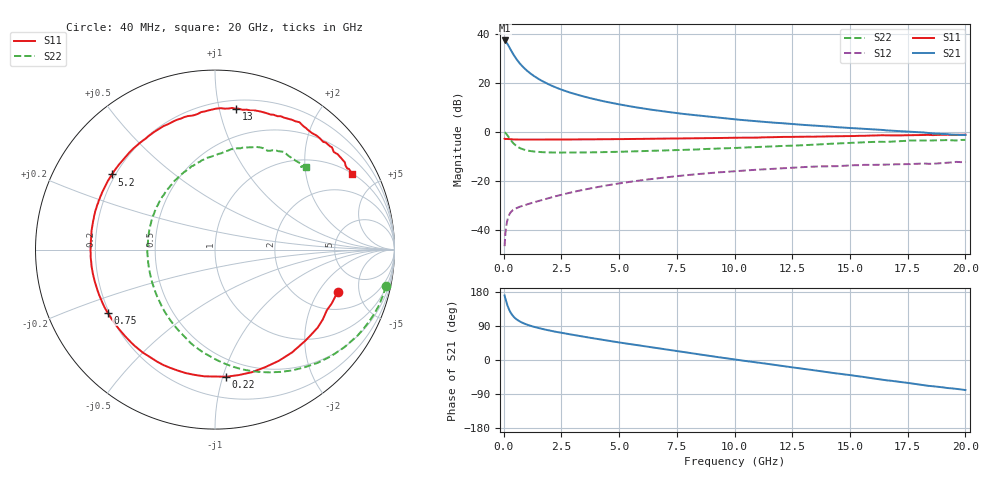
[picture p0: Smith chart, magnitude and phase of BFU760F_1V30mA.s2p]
! Filename:  P:\Prog\Test\Noise\ATS_data\Testdata_Net\Split files Spar\BFU760F_2W_C1_1V_5mA_60mA_Bias7_D.s2p
! Date/Time: Mon 06/Feb/2012 15:06:17
! BFU760_2W_C1_1V_5mA_60mA_Bias7_R.s2p
! MDIF S-parameter v. bias file
! BFU760_2W_C1_1V_5mA_60mA
! Date/time Fri Mar 18 10:56:44 2011
! VAR V_out= 1.0002
! VAR I_out= 30.0000
! VAR V_in= 0.8043
! VAR I_in= 0.0968
! Device data file deembeded for feedlines and parallel
! Original file: \Split files Spar\BFU760_2W_C1_1V_5mA_60mA_Bias7_R.s2p
! Feed-files: PR003V01_101208_Feed1.s2p, PR003V01_101208_Feed2.s2p
! Parallel-file: PR003V01_101208_Par.s2p
# MHz S MA R 50
!  Freq-MHz  S11-mag  S11-arg  S21-mag  S21-arg  S12-mag  S12-arg  S22-mag  S22-arg
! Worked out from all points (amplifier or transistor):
!   167 points, 40 MHz to 20 GHz, reference 50 ohm
!   highest |S21| = 37.4 dB at 40 MHz (marker M1)
!   |S21| within 3 dB of that: start of sweep to 257.1 MHz
!   unconditionally stable (mu >= 1): 3.655 GHz to 15.18 GHz
!   at 550 MHz: K = 0.35, MSG = 30.5 dB, |S12| = -31.2 dB
!   at 4.2 GHz: K = 1.02, MAG = 16.7 dB, |S12| = -22.4 dB
!   at 20 GHz: K = 0.94, MSG = 5.5 dB, |S12| = -12.4 dB
!   S11 on the Smith chart (normalised r, x): 40 MHz: 3.05, -3.02; 220 MHz: 0.36, -1.03; 750 MHz: 0.19, -0.26; 5.2 GHz: 0.19, +0.32; 13 GHz: 0.27, +1.13; 20 GHz: 1.01, +3.60
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40  0.7225 -19.1  73.75 170.3  0.004595 81.9  0.9745 -12.0
50  0.7163 -24.7  72.94 167.1  0.005339 77.6  0.9695 -15.6
60  0.709 -28.5  70.35 164.8  0.006654 79.4  0.9653 -18.7
80  0.7184 -37.2  71.25 160.3  0.008843 74.3  0.9475 -25.1
120  0.7159 -53.2  67.52 151.7  0.01255 67.5  0.9029 -37.1
160  0.7123 -67.1  62.89 144.3  0.01568 61.4  0.8516 -47.8
220  0.711 -84.9  56.37 135.0  0.01926 54.4  0.7725 -61.9
300  0.707 -103.4  47.79 125.2  0.02246 47.7  0.6839 -77.3
420  0.6996 -122.7  38.21 115.1  0.02547 41.9  0.5835 -95.0
550  0.6955 -136.3  30.85 107.6  0.0275 39.0  0.5131 -109.5
750  0.694 -149.6  23.47 100.1  0.03001 37.5  0.4553 -125.5
1150  0.6931 -165.0  15.7 90.5  0.0344 38.7  0.4052 -145.9
1650  0.694 -176.3  11.05 82.3  0.04036 41.3  0.3844 -161.3
2350  0.6936 173.3  7.752 73.4  0.04942 43.1  0.377 -175.1
3400  0.7003 161.2  5.377 62.3  0.06452 42.8  0.3784 170.4
5200  0.7107 143.9  3.498 44.5  0.09118 36.9  0.3932 151.2
6800  0.7222 130.2  2.667 29.8  0.1142 29.0  0.4127 136.6
10200  0.758 102.9  1.766 -0.2  0.1588 8.6  0.4735 108.8
13000  0.7938 81.4  1.384 -23.5  0.1901 -9.7  0.5337 87.9
13400  0.7939 78.8  1.345 -26.8  0.1939 -12.8  0.5445 85.0
16800  0.8457 53.3  1.053 -54.9  0.215 -34.7  0.6307 60.8
20000  0.8729 29.0  0.8604 -79.4  0.2403 -56.0  0.6851 42.3
